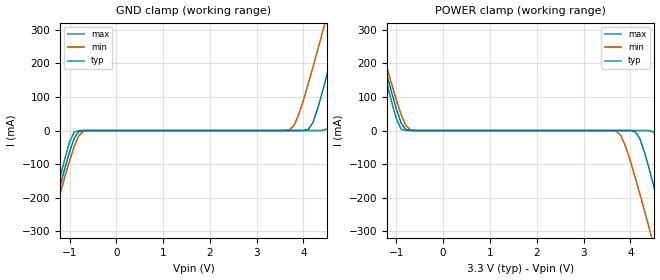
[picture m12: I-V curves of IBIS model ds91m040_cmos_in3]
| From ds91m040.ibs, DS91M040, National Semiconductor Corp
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|   Model  ds91m040_cmos_in3
[Model]   ds91m040_cmos_in3
Model_type Input
Vinh=2.0
Vinl=0.8
|   Typ   Min   Max
C_comp   2.03pF   2.00pF   2.06pF
[Model Spec]
S_overshoot_high   3.3   3.0   3.6
S_overshoot_low   0.0   0.0   0.0
[Temperature Range]   25   85   -40
[Voltage Range]   3.3   3.0   3.6
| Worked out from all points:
|   GND clamp passes 1 mA (typ) near -0.73 V on its own axis
|   POWER clamp passes 1 mA (typ) near -0.73 V on its own axis
[GND Clamp]
-3.3V     -1.35A     -1.302A    -1.413A
-1.5V     -327.7mA   -340.2mA   -314.7mA
-1.4V     -272.6mA   -288.4mA   -255.4mA
-900mV    -23.1mA    -47.78mA   -4.26mA
-600mV    -3.125uA   -136.6uA   -6.954nA
3.7V      2.203nA    2.208mA    7.652pA
3.9V      3.125uA    47.78mA    8.558pA
4.2V      23.1mA     186.8mA    6.954nA
4.5V      164.6mA    340.2mA    4.26mA
4.8V      327.7mA    497.7mA    139.4mA
5.1V      495.3mA    657mA      314.7mA
6.5V      1.293A     1.41A      1.167A
[POWER Clamp]
-3.3V     1.35A      1.302A     1.228A
-1.5V     327.7mA    340.2mA    314.7mA
-1.4V     272.6mA    288.4mA    255.4mA
-900mV    23.1mA     47.78mA    4.26mA
-600mV    3.125uA    136.6uA    6.954nA
3.7V      -2.203nA   -2.208mA   -7.653pA
3.9V      -3.125uA   -47.78mA   -8.558pA
4.2V      -23.1mA    -186.8mA   -6.954nA
4.5V      -164.6mA   -340.2mA   -4.26mA
4.8V      -327.7mA   -497.7mA   -139.4mA
5.1V      -495.3mA   -657mA     -314.7mA
6.5V      -1.293A    -1.302A    -1.167A
